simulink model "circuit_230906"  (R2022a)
settings: Solver=VariableStepAuto  StartTime=0.0  StopTime=1e-4  RelTol=1e-3  AbsTol=1e-3
libraries: fl_lib x11, nesl_utility x3, ee_lib x1

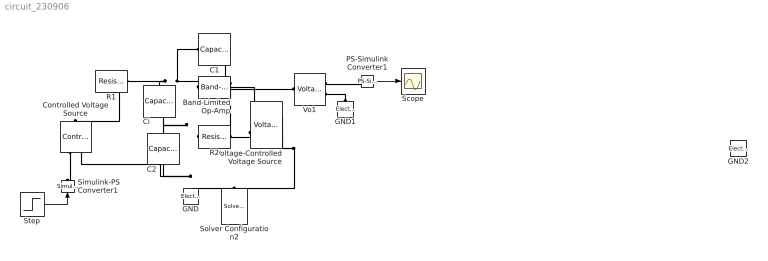
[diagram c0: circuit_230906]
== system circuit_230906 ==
  Band-Limited Op-Amp : ee_lib/Integrated Circuits/Band-Limited Op-Amp  A=1e6  Rin=1e7 Ohm  Rout=0 Ohm  Vmin=-15 V  Vmax=15 V  Vdotmax=1e8 V/s  f=10 Hz  V0=0 V
  C1 : fl_lib/Electrical/Electrical Elements/Capacitor  c=1e-11 F  r=0 Ohm  g=1e-6 1/Ohm  i_specify=off  i_priority=None  i=0 A  i_nominal_specify=off  i_nominal_unit=A  i_nominal_value=1  v_specify=off  v_priority=None  v=0 V  v_nominal_specify=off  v_nominal_unit=V  v_nominal_value=1  vc_specify=off  vc_priority=High  vc=0 V  vc_nominal_specify=off  vc_nominal_unit=V  vc_nominal_value=1
  C2 : fl_lib/Electrical/Electrical Elements/Capacitor  c=1e-11 F  r=0 Ohm  g=1e-6 1/Ohm  i_specify=off  i_priority=None  i=0 A  i_nominal_specify=off  i_nominal_unit=A  i_nominal_value=1  v_specify=off  v_priority=None  v=0 V  v_nominal_specify=off  v_nominal_unit=V  v_nominal_value=1  vc_specify=off  vc_priority=High  vc=0 V  vc_nominal_specify=off  vc_nominal_unit=V  vc_nominal_value=1
  Ci : fl_lib/Electrical/Electrical Elements/Capacitor  c=1e-12 F  r=1e-6 Ohm  g=0 1/Ohm  i_specify=off  i_priority=None  i=0 A  i_nominal_specify=off  i_nominal_unit=A  i_nominal_value=1  v_specify=off  v_priority=None  v=0 V  v_nominal_specify=off  v_nominal_unit=V  v_nominal_value=1  vc_specify=off  vc_priority=High  vc=0 V  vc_nominal_specify=off  vc_nominal_unit=V  vc_nominal_value=1
  Controlled Voltage Source : fl_lib/Electrical/Electrical Sources/Controlled Voltage Source
  GND : fl_lib/Electrical/Electrical Elements/Electrical Reference
  GND1 : fl_lib/Electrical/Electrical Elements/Electrical Reference
  GND2 : fl_lib/Electrical/Electrical Elements/Electrical Reference
  PS-Simulink Converter1 : nesl_utility/PS-Simulink Converter  PhysicalDomain=network_engine_domain  SubClassName=ps_output  LeftPortType=input  RightPortType=output  PseudoPeriodic=off  Frequencies=[]  VectorFormat=1-D array  Unit=inherit  AffineConversion=off
  R1 : fl_lib/Electrical/Electrical Elements/Resistor  R=200 kOhm  i_specify=off  i_priority=None  i=0 A  i_nominal_specify=off  i_nominal_unit=A  i_nominal_value=1  v_specify=off  v_priority=None  v=0 V  v_nominal_specify=off  v_nominal_unit=V  v_nominal_value=1
  R2 : fl_lib/Electrical/Electrical Elements/Resistor  R=200 kOhm  i_specify=off  i_priority=None  i=0 A  i_nominal_specify=off  i_nominal_unit=A  i_nominal_value=1  v_specify=off  v_priority=None  v=0 V  v_nominal_specify=off  v_nominal_unit=V  v_nominal_value=1
  Scope : Scope
  Simulink-PS Converter1 : nesl_utility/Simulink-PS Converter  PhysicalDomain=network_engine_domain  SubClassName=ps_input  LeftPortType=input  RightPortType=output  PseudoPeriodic=off  Frequencies=[]  NoiseDistribution=none  NoiseParameters=[]  Unit=1  AffineConversion=off  FilteringAndDerivatives=provide  SimscapeFilterOrder=1  InputFilterTimeConstant=0.001  UdotUserProvided=0
  Solver Configuration2 : nesl_utility/Solver Configuration  PhysicalDomain=network_engine_domain  SubClassName=solver  LeftPortType=input  RightPortType=generic  Tones=[]  Harmonics=[]  SimulateNoise=off  Profile=off  UseLocalSampling=off  EnableSwitchedLinearOptims=on  FrequencyDomain=off  UseCCode=off  RelTol=0.001  AbsTol=1e-06  MinStep=1e-09  ToWorkspace=off  RevertToSquareIcSolve=off  NumHomotopyIterations=100  PhasorMode=off  PhasorModeNumHarmonics=1  IndexReductionMethod=DerivativeReplacement  DoDC=off  ResidualTolerance=1e-09  UseLocalSolver=off  LocalSolverChoice=NE_BACKWARD_EULER_ADVANCER  LocalSolverSampleTime=0.001  DoFixedCost=off  MaxNonlinIter=3  MaxModeIter=2  ComputeImpulses=off  ImpulseIterations=2  LinearAlgebra=Sparse  LinearAlgebraNumThread=0  EquationFormulation=NE_TIME_EF  DelaysMemoryBudget=1024  AutomaticFiltering=on  FilteringTimeConstant=0.001  PartitionStorageMethod=AS_NEEDED  PartitionMemoryBudget=1024  PartitionMethod=FAST
  Step : Step  Time=0  SampleTime=0
  Vo1 : fl_lib/Electrical/Electrical Sensors/Voltage Sensor
  Voltage-Controlled Voltage Source : fl_lib/Electrical/Electrical Sources/Voltage-Controlled Voltage Source  K=-1  v1_specify=off  v1_priority=None  v1=0 V  v1_nominal_specify=off  v1_nominal_unit=V  v1_nominal_value=1  v2_specify=off  v2_priority=None  v2=0 V  v2_nominal_specify=off  v2_nominal_unit=V  v2_nominal_value=1
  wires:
  Step/1 -> Simulink-PS Converter1/1
  PS-Simulink Converter1/1 -> Scope/1
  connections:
  Controlled Voltage Source/RConn1 -- Simulink-PS Converter1/RConn1
  C1/RConn1 -- R1/LConn1 -- Ci/LConn1 -- Band-Limited Op-Amp/LConn2
  GND1/LConn1 -- Vo1/RConn2
  PS-Simulink Converter1/LConn1 -- Vo1/RConn1
  R2/RConn1 -- C2/LConn1 -- Ci/RConn1 -- Band-Limited Op-Amp/LConn1
  Band-Limited Op-Amp/RConn1 -- Voltage-Controlled Voltage Source/LConn1 -- C1/LConn1 -- Vo1/LConn1
  Solver Configuration2/RConn1 -- Controlled Voltage Source/RConn2 -- C2/RConn1 -- GND/LConn1 -- Voltage-Controlled Voltage Source/RConn1 -- Voltage-Controlled Voltage Source/RConn2
  Voltage-Controlled Voltage Source/LConn2 -- R2/LConn1
  R1/RConn1 -- Controlled Voltage Source/LConn1
